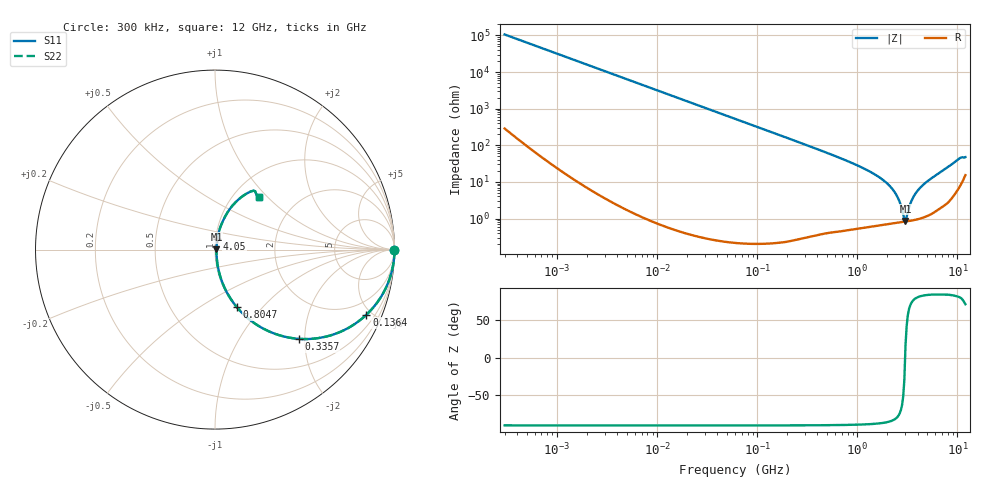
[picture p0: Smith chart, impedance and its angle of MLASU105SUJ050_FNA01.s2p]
! MLASU105SUJ050_FNA01  S-PARAMETER MODEL  ( General Type )
! Model Generated by TAIYO YUDEN Corporation (http://www.ty-top.com)
! Version 2.0
! TAIYO YUDEN Control No. 120810
! Copyright(c) 2011 TAIYO YUDEN CO.,LTD. All Rights Reserved.
! Product Description (link to TY-COMPAS)
! https://ds.yuden.co.jp/TYCOMPAS/or/detail?pn=MLASU105SUJ050CFNA01&u=M
! Products Name : Multilayer Ceramic Capacitors
! Characteristics :
!  Capacitance : 5 pF , Rated Voltage : 50V , TCC : UJ / U2J
!  Case Size : 1.0 x 0.5 / 0.039 x 0.02 [mm/inch] , Thickness : 0.5 / 0.02 [mm/inch]
!  (Conditions: Temperature = 25 degC , DC Bias Current/Voltage = 0A / 0V)
! External Node Assignments :
!  1  o---| |---o  2
! GND o---------o GND
! Frequency Range : 0.3MHz  -  12000MHz  [ 401 STEP ]
# MHz S RI R 50
! Freq[MHz].  S11 Real  S11 Imag  S21 Real  S21 Imag  S12 Real  S12 Imag  S22 Real  S22 Imag
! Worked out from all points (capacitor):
!   401 points, 300 kHz to 12 GHz, reference 50 ohm
!   read as one part in series: C = 5.01 pF near 316.3 kHz
!   lowest |Z| = 856 mohm at 3.026 GHz (marker M1)
!   series resonance near 3 GHz, so ESL is about 560 pH
!   S11 on the Smith chart (normalised r, x): 300 kHz: open; 136.4 MHz: 1.00, -4.65; 335.7 MHz: 1.01, -1.87; 804.7 MHz: 1.01, -0.73; 4.05 GHz: 1.02, +0.12; 12 GHz: 1.31, +0.90
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0.3  1 -0.000945  3.45e-06 0.000945  3.45e-06 0.000945  1 -0.000945
1.769972  1 -0.00557  3.37e-05 0.00557  3.37e-05 0.00557  1 -0.00557
10.44266  0.9989 -0.0329  0.00109 0.0329  0.00109 0.0329  0.9989 -0.0329
60  0.9654 -0.1825  0.0346 0.1825  0.0346 0.1825  0.9654 -0.1825
136.3989  0.8434 -0.3629  0.1566 0.3629  0.1566 0.3629  0.8434 -0.3629
225.6362  0.6616 -0.4723  0.3384 0.4723  0.3384 0.4723  0.6616 -0.4723
335.7268  0.466 -0.4971  0.534 0.4971  0.534 0.4971  0.466 -0.4971
353.9943  0.4392 -0.4944  0.5608 0.4944  0.5608 0.4944  0.4392 -0.4944
804.7407  0.1215 -0.3203  0.8785 0.3203  0.8785 0.3203  0.1215 -0.3203
1441.349  0.0336 -0.1631  0.9664 0.1631  0.9664 0.1631  0.0336 -0.1631
2088.533  0.0131 -0.0773  0.9869 0.0773  0.9869 0.0773  0.0131 -0.0773
2514.07  0.00901 -0.0376  0.991 0.0376  0.991 0.0376  0.00901 -0.0376
2650.866  0.00846 -0.0265  0.9915 0.0265  0.9915 0.0265  0.00846 -0.0265
2870.14  0.00811 -0.00994  0.9919 0.00994  0.9919 0.00994  0.00811 -0.00994
3026.31  0.00818 0.00228  0.9918 -0.00228  0.9918 -0.00228  0.00818 0.00228
3107.553  0.00833 0.00736  0.9917 -0.00736  0.9917 -0.00736  0.00833 0.00736
3547.679  0.00986 0.0324  0.9901 -0.0324  0.9901 -0.0324  0.00986 0.0324
4050.141  0.0129 0.0579  0.9871 -0.0579  0.9871 -0.0579  0.0129 0.0579
5278.635  0.025 0.111  0.975 -0.111  0.975 -0.111  0.025 0.111
7648.807  0.0703 0.2083  0.9297 -0.2083  0.9297 -0.2083  0.0703 0.2083
9708.23  0.1547 0.2981  0.8453 -0.2981  0.8453 -0.2981  0.1547 0.2981
12000  0.2466 0.2931  0.7534 -0.2931  0.7534 -0.2931  0.2466 0.2931
